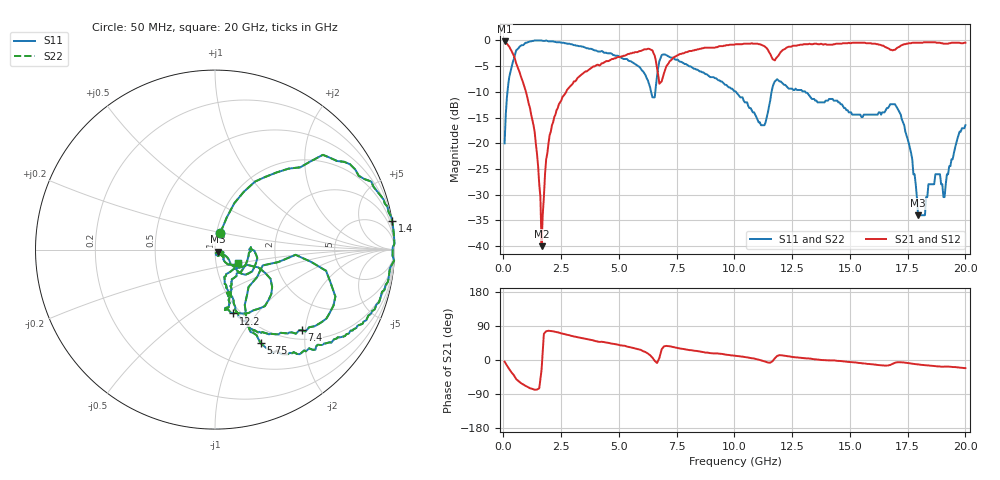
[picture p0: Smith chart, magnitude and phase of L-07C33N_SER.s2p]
#	mhz	s	ma	r	50
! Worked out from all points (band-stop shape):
!   400 points, 50 MHz to 20 GHz, reference 50 ohm
!   highest |S21| = -0.18 dB at 50 MHz (marker M1); lowest = -40.0 dB at 1.65 GHz (marker M2)
!   |S21| within 3 dB of the highest: 7.419 GHz to 11.61 GHz (4.189 GHz wide, 44 % of centre); 11.86 GHz to end of sweep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
!   lowest |S11| = -34.0 dB at 17.95 GHz (marker M3), VSWR 1.04, Z = 51.7 - j1.14 ohm
!   |S11| at or under -10 dB: 6.392 GHz to 6.574 GHz (182.4 MHz wide, 2.81 % of centre); 10.07 GHz to 11.61 GHz (1.54 GHz wide, 14.2 % of centre); 13.07 GHz to end of sweep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
!   |S22| runs from -34.0 to 0.0 dB; largest |S21 - S12| = 0
!   S11 on the Smith chart (normalised r, x): 50 MHz: 1.04, +0.20; 1.4 GHz: 0, +12; 5.75 GHz: 0.80, -1.26; 7.4 GHz: 1.20, -1.92; 12.2 GHz: 0.93, -0.76; 20 GHz: 1.28, -0.20
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50  0.1 72.3  0.98 -4.3  0.98 -4.3  0.1 72.3
200  0.36 63.5  0.9 -19.4  0.9 -19.4  0.36 63.5
550  0.8 41.3  0.6 -50.3  0.6 -50.3  0.8 41.3
1400  1 9.2  0.1 -78.2  0.1 -78.2  1 9.2
1650  1 1.8  0.01 -26.1  0.01 -26.1  1 1.8
1850  1 -3.5  0.07 76.0  0.07 76.0  1 -3.5
2100  0.98 -9.5  0.15 76.1  0.15 76.1  0.98 -9.5
3400  0.87 -32.9  0.47 57.7  0.47 57.7  0.87 -32.9
5750  0.58 -63.9  0.77 29.8  0.77 29.8  0.58 -63.9
6450  0.28 -48.1  0.8 6.1  0.8 6.1  0.28 -48.1
6700  0.54 -7.3  0.46 -1.3  0.46 -1.3  0.54 -7.3
7400  0.66 -42.9  0.69 33.6  0.69 33.6  0.66 -42.9
10050  0.32 -70.9  0.92 11.0  0.92 11.0  0.32 -70.9
11300  0.15 -46.6  0.88 -3.9  0.88 -3.9  0.15 -46.6
12200  0.37 -74.0  0.83 11.0  0.83 11.0  0.37 -74.0
13350  0.27 -71.5  0.92 3.0  0.92 3.0  0.27 -71.5
16700  0.23 -6.7  0.83 -13.7  0.83 -13.7  0.23 -6.7
17350  0.15 -41.8  0.92 -6.7  0.92 -6.7  0.15 -41.8
17950  0.02 -33.3  0.95 -11.6  0.95 -11.6  0.02 -33.3
18700  0.05 -27.7  0.96 -16.2  0.96 -16.2  0.05 -27.7
19100  0.03 -21.2  0.93 -17.4  0.93 -17.4  0.03 -21.2
20000  0.15 -30.2  0.95 -21.5  0.95 -21.5  0.15 -30.2
